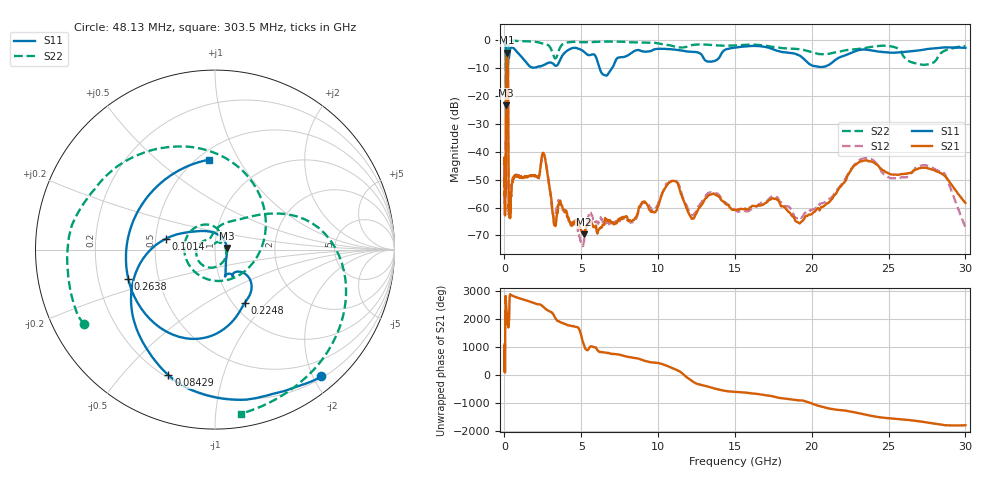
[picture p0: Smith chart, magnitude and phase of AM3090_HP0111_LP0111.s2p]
! Date/Time: Thu, Feb 28, 2019 2:01 PM
! Network Analyzer: Agilent Technologies E8364B Rev: A.07.50.67
! Sweep from 0.010 to 30.000 GHz, 1601 Points, Sweep Type: LOG
! Power Supply: 5.023 V, 0.002 A
# Hz S DB R 50
!freq MagS11 AngS11 MagS21 AngS21 MagS12 AngS12 MagS22 AngS22
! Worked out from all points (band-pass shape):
!   1601 points, 10 MHz to 30 GHz, reference 50 ohm
!   highest |S21| = -4.53 dB at 159.9 MHz (marker M1); lowest = -69.6 dB at 5.154 GHz (marker M2)
!   |S21| within 3 dB of the highest: 113.9 MHz to 218 MHz (104.1 MHz wide, 62.7 % of centre)
!   lowest |S11| = -23.4 dB at 109.9 MHz (marker M3), VSWR 1.14, Z = 57.1 + j1.11 ohm
!   |S11| at or under -10 dB: 100.8 MHz to 218.2 MHz (117.5 MHz wide, 73.6 % of centre); 6.184 GHz to 7.011 GHz (826.9 MHz wide, 12.5 % of centre)
!   |S22| runs from -30.9 to -0.2 dB; largest |S21 - S12| = 0.012
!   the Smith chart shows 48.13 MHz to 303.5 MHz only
!   S11 on the Smith chart (normalised r, x): 48.13 MHz: 0.23, -2.12; 84.29 MHz: 0.21, -0.67; 101.4 MHz: 0.56, +0.07; 224.8 MHz: 1.12, -0.76; 263.8 MHz: 0.33, -0.14; 303.5 MHz: 0.57, +0.76
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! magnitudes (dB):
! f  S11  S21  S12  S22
! 10 MHz  -0.2  -44.4  -45.8  -0.6
! 38.04 MHz  -0.5  -59.2  -62.6  -1.4
! 48.13 MHz  -0.7  -50.3  -50.4  -1.5
! 84.29 MHz  -2.5  -52.9  -52.6  -5.1
! 101.4 MHz  -11.0  -17.9  -17.9  -15.4
! 109.9 MHz  -23.4  -9.1  -9.1  -15.5
! 144.7 MHz  -16.2  -4.7  -4.7  -26.3
! 159.9 MHz  -15.8  -4.5  -4.5  -21.7
! 224.8 MHz  -9.3  -9.2  -9.2  -13.4
! 263.8 MHz  -5.9  -50.5  -51.4  -1.7
! 303.5 MHz  -6.0  -60.6  -61.8  -0.7
! 550.5 MHz  -2.8  -49.6  -49.7  -0.3
! 2.084 GHz  -9.8  -48.8  -49.0  -0.7
! 2.558 GHz  -9.0  -40.7  -40.7  -1.3
! 3.236 GHz  -8.9  -66.3  -64.0  -6.3
! 5.154 GHz  -4.1  -69.6  -72.6  -0.8
! 7.926 GHz  -5.8  -63.3  -64.6  -0.7
! 10.92 GHz  -3.3  -50.5  -50.4  -2.1
! 19.41 GHz  -6.4  -64.7  -63.2  -3.5
! 23.48 GHz  -3.4  -43.1  -42.3  -2.9
! 27.83 GHz  -3.1  -46.4  -45.7  -8.3
! 30 GHz  -2.8  -58.3  -67.0  -2.2
